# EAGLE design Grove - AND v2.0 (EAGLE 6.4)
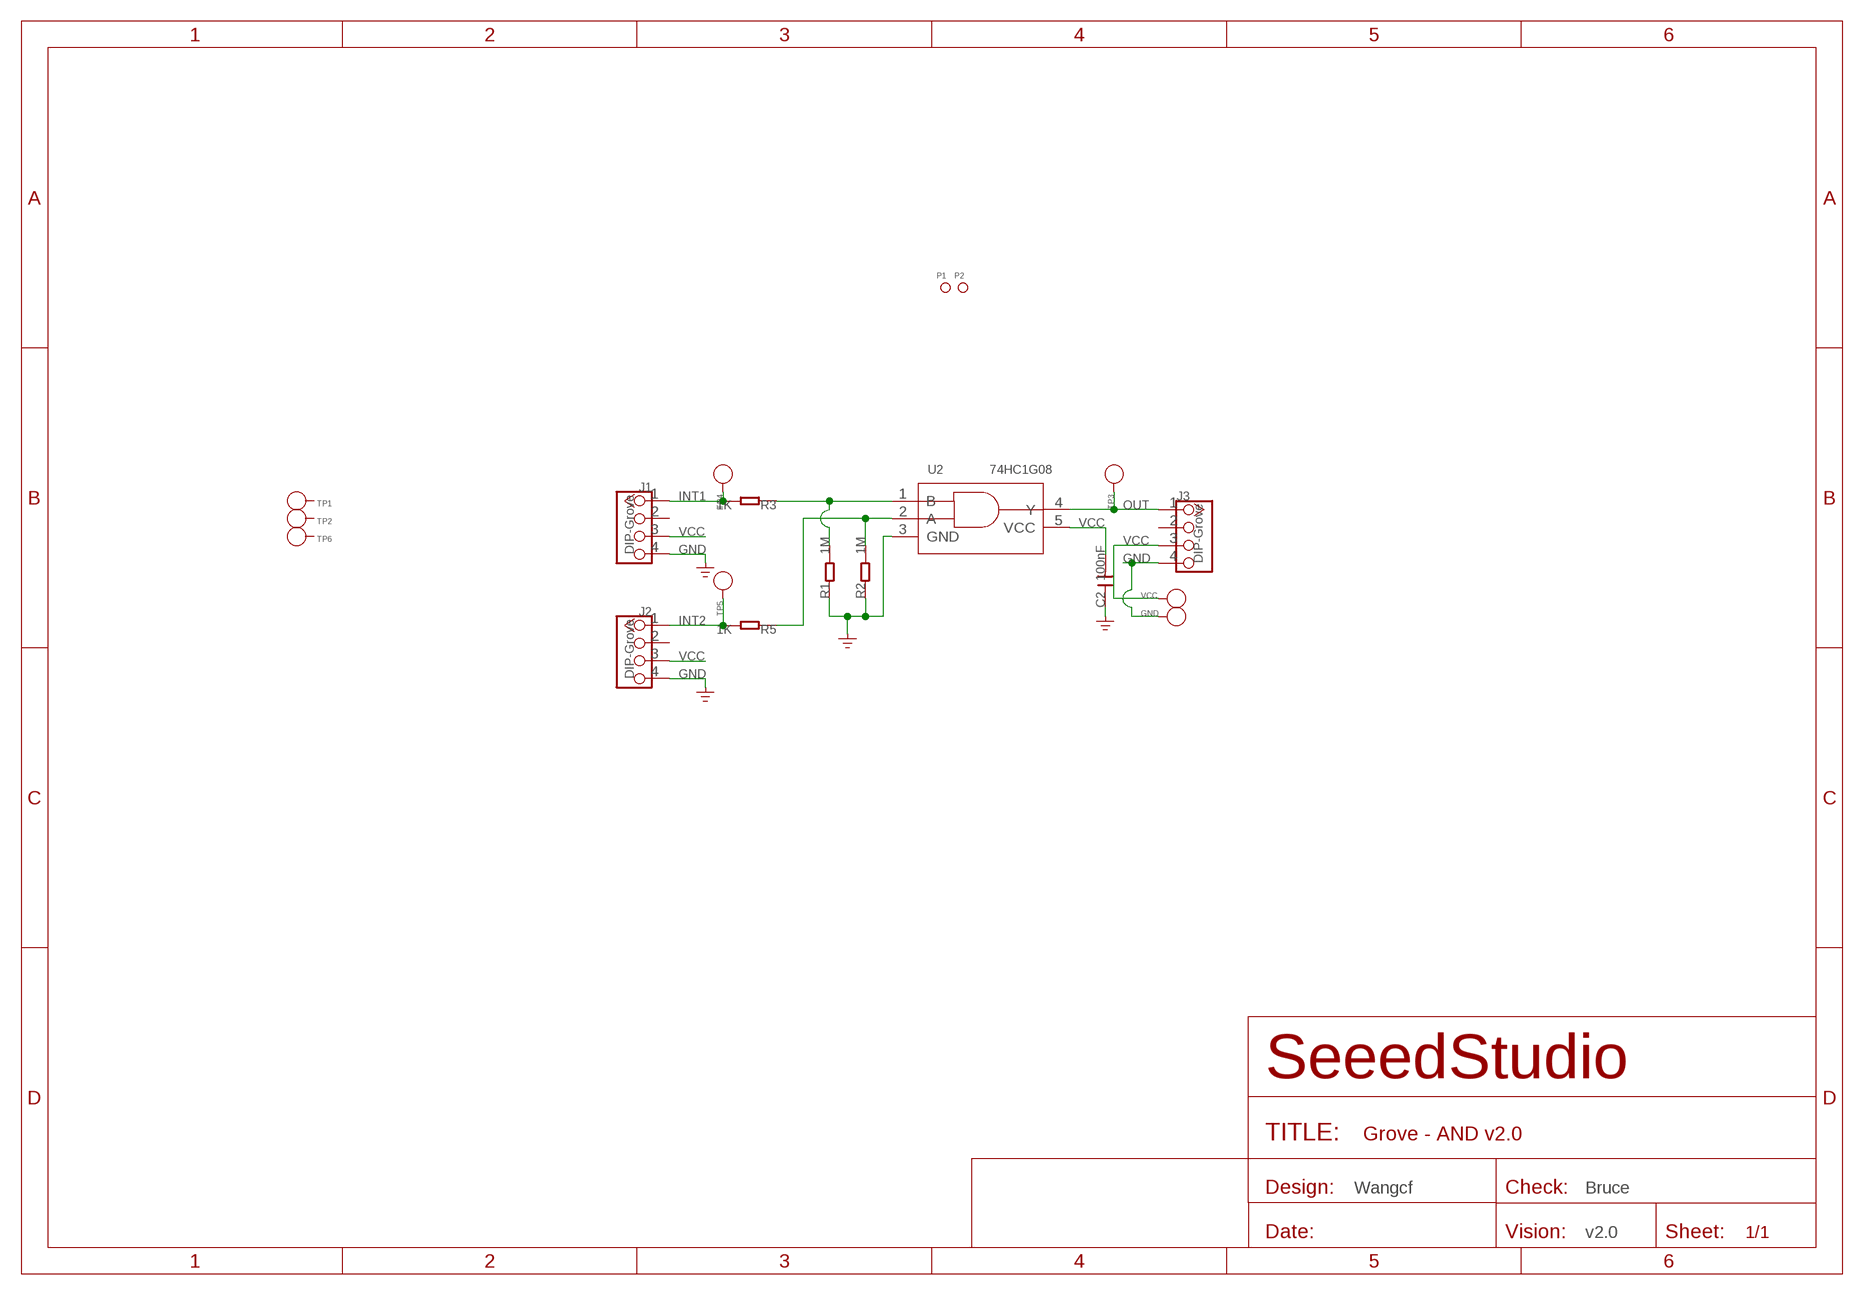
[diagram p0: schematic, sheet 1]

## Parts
C2  100nF  C-0603  [C0603]
GND  PAD-TEST-POINT'4545'  [TP_4545]
J1  DIP-Grove  TWIG-4P-2.0-2.0  [4P-2.0]
J2  DIP-Grove  TWIG-4P-2.0-2.0  [4P-2.0]
J3  DIP-Grove  TWIG-4P-2.0-2.0  [4P-2.0]
P1  PAD-MARK  [ROUND-MARK-1.0]
P2  PAD-MARK  [ROUND-MARK-1.0]
R1  1M  R-0603  [R0603]
R2  1M  R-0603  [R0603]
R3  1K  R-0603  [R0603]
R5  1K  R-0603  [R0603]
TP1  PAD-TEST-POINT'4545'  [TP_4545]
TP2  PAD-TEST-POINT'4545'  [TP_4545]
TP3  PAD-TEST-POINT'4545'  [TP_4545]
TP4  PAD-TEST-POINT'4545'  [TP_4545]
TP5  PAD-TEST-POINT'4545'  [TP_4545]
TP6  PAD-TEST-POINT'4545'  [TP_4545]
U2  74HC1G08  74HC1G08'GW'  [SOT-353]
VCC  PAD-TEST-POINT'4545'  [TP_4545]

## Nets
GND: C2.1 GND.T J1.4 J2.4 J3.4 R1.1 R2.1 U2.3(GND)
INT1: J1.1 R3.2 TP4.T
INT2: J2.1 R5.2 TP5.T
N$2: R1.2 R3.1 U2.1(B)
N$5: R2.2 R5.1 U2.2(A)
OUT: J3.1 TP3.T U2.4(Y)
VCC: C2.2 J1.3 J2.3 J3.3 U2.5(VCC) VCC.T
Unconnected: J1.2 J2.2 J3.2 TP1.T TP2.T TP6.T

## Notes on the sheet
- Wangcf | Bruce
- v2.0

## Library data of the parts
C2 = Discrete:C*: Ceramic Capacitors
GND TP1-TP6 VCC = Discrete:PAD-TEST-POINT; PARTNO: DNP
J1-J3 = Connector :TWIG-4P-2.0
P1 P2 = Discrete:PAD-MARK; PARTNO: DNP
R1-R3 R5 = Discrete:R*
U2 = template:74HC1G08: 2-input AND gate

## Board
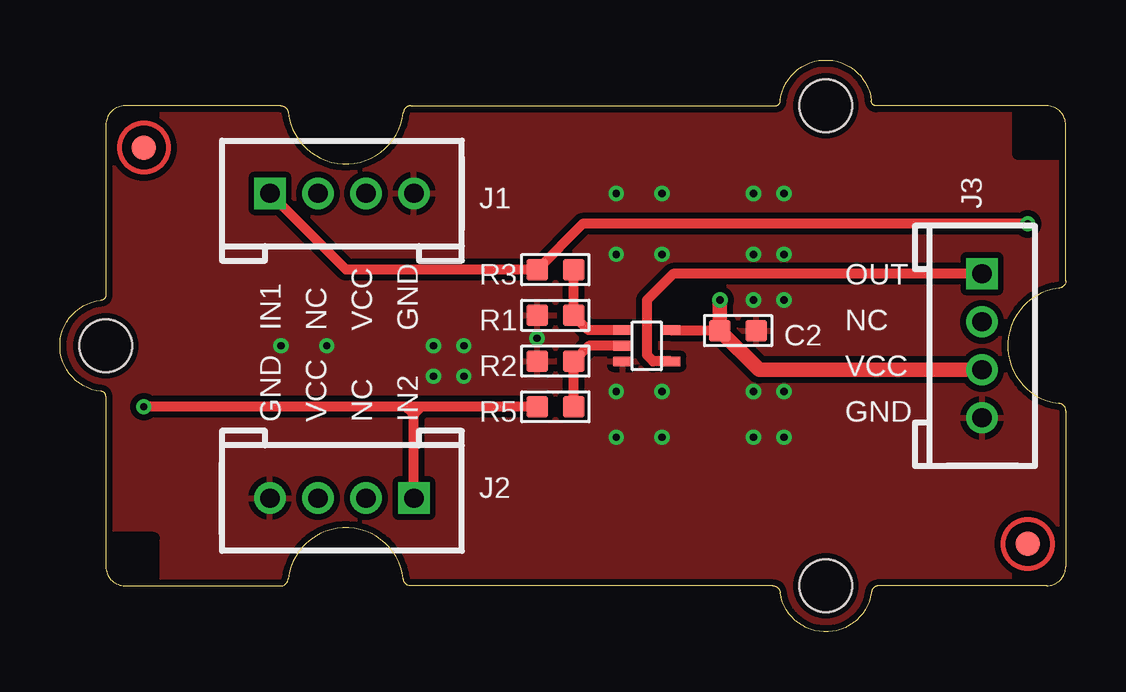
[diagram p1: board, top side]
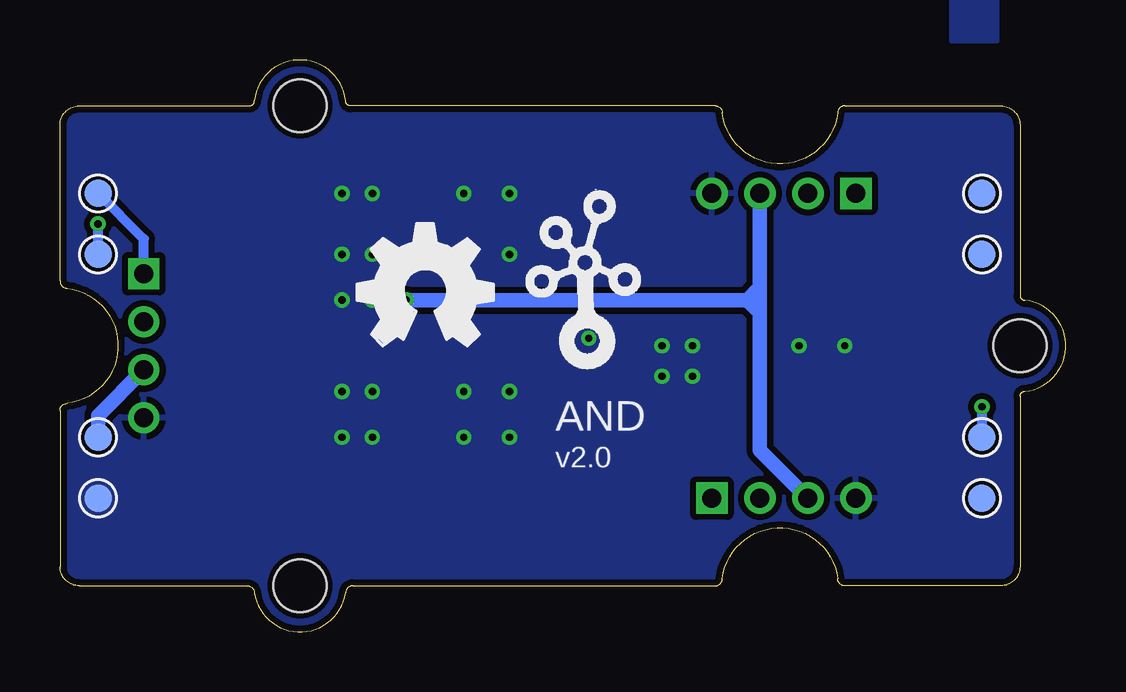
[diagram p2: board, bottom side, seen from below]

Size 41.91 x 23.83 mm. Coordinates in mm from the lower left corner, seen from the top.
Copper layers (1*16): Top 0.035mm / dielectric 1.5mm / Bottom 0.035mm
Design rules "SeeedStudio_DRU_no_angle_20130527 *": minimum track width 6mil, minimum drill 12mil, track to track 6mil, track to pad 6mil, pad to pad 6mil, via to via 6mil, smd to smd 0mil, copper to edge 10mil, drill to drill 10mil, minimum pad ring 10mil, minimum via ring 6mil, stop-mask expansion 2mil, vias tented up to drill 25mil, thermal gap 10mil

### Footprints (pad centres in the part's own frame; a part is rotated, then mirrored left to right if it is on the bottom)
C0603 = smd 0.889 x 0.889: 1 -0.762,0; 2 0.762,0
TP_4545 = smd 1.143 x 1.143: T 0,0
4P-2.0 = drill 0.8 pad 1.27 square: 1 -3,0 | drill 0.8 pad 1.27: 2 -1,0; 3 1,0; 4 3,0
ROUND-MARK-1.0 = smd 1.016 x 1.016: P$1 0,0
R0603 = smd 0.889 x 0.889: 1 -0.762,0; 2 0.762,0
SOT-353 = smd 0.4 x 0.8: 1 -0.65,-1; 2 0,-1; 3 0.65,-1; 4 0.65,1; 5 -0.65,1
GROVE-3CONNECTOR-FIRST = hole 2.2: -10,-10; -10,10; 20,0

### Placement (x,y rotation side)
C2  28.26,12.56 180 top
GND  40.32,5.57 0 bottom
J1  11.75,18.27 0 top
J2  11.75,5.57 180 top
J3  38.42,11.92 270 top
P1  3.49,20.18 0 top
P2  40.32,3.67 0 top
R1  20.64,13.19 0 top
R2  20.64,11.29 0 top
R3  20.64,15.1 180 top
R5  20.64,9.38 180 top
TP1  3.49,18.27 0 bottom
TP2  3.49,15.73 0 bottom
TP3  40.32,18.27 0 bottom
TP4  40.32,15.73 0 bottom
TP5  3.49,8.11 0 bottom
TP6  3.49,5.57 0 bottom
U2  24.45,11.92 270 top
U$2  [GROVE-3CONNECTOR-FIRST]  21.91,11.92 180 top
U$4  [OSHW_FILLX200_NOTEXT]  29.53,11.92 0 bottom
U$8  [TWIGLOGO]  20,11.92 0 bottom
VCC  40.32,8.11 0 bottom

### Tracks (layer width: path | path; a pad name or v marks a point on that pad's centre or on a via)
GND  (via drill 0.3 pad 0.64)
  other vias: 28.89,13.83 23.18,15.73 25.08,15.73 28.89,15.73 23.18,10.02 15.56,11.92 25.08,10.02 16.83,11.92 19.88,12.24 30.16,13.83 30.16,15.73 30.16,10.02 28.89,10.02 23.18,8.11 25.08,8.11 11.11,11.92 9.21,11.92 23.18,18.27 25.08,18.27 28.89,18.27 30.16,18.27 28.89,8.11 30.16,8.11 16.83,10.65 15.56,10.65
  pour Bottom: 2.86,26.53 4.76,26.53 4.76,24.62 2.86,24.62
  pour Bottom (isolate 0.254): 0.32,23.99 42.23,23.99 42.23,-0.14 -0.32,-0.14 -0.32,23.99
  pour Top (isolate 0.254): 0.32,23.99 42.23,23.99 42.23,-0.14 -0.32,-0.14 -0.32,23.99
INT1  (via drill 0.3 pad 0.64)
  Top 0.406: J1.1 11.92,15.1 R3.2 21.78,17 v40.32,17
  Bottom 0.406: TP4.T v40.32,17
INT2  (via drill 0.3 pad 0.64)
  Top 0.406: R5.2 15.05,9.38 | 15.05,9.38 14.67,9.38 | 14.67,9.38 14.42,9.38 | 14.42,9.38 v3.49,9.38 | J2.1 14.75,9.01 14.75,9.08 | 14.75,9.08 14.75,9.3 14.67,9.38 | 14.42,9.38 14.67,9.13 | 14.75,9.08 15.05,9.38
  Bottom 0.406: v3.49,9.38 TP5.T
N$2
  Top 0.406: U2.1 22.02,12.57 R1.2 R3.1
N$5
  Top 0.406: U2.2 22.04,11.92 R2.2 R5.1
OUT
  Top 0.406: J3.1 25.54,14.92 24.45,13.83 24.45,11.54 24.72,11.27 U2.4
  Bottom 0.406: J3.1 38.42,16.37 TP3.T
VCC  (via drill 0.3 pad 0.64)
  Top 0.406: U2.5 27.48,12.57 C2.2
  Top 0.61: J3.3 29.13,10.92 C2.2 v27.5,13.83
  Bottom 0.61: 12.75,13.83 12.75,7.57 J2.3 | J1.3 12.75,13.83 | VCC.T 40.32,9.02 J3.3 | v27.5,13.83 13.27,13.83 | 13.27,13.83 12.75,13.83 | 13.27,13.83 12.76,13.32 12.76,14.33 13.27,13.83

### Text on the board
tPlace: OUT | IN1 | NC | VCC | GND | NC | VCC | GND | VCC | NC | IN2 | GND
bPlace: AND | v2.0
